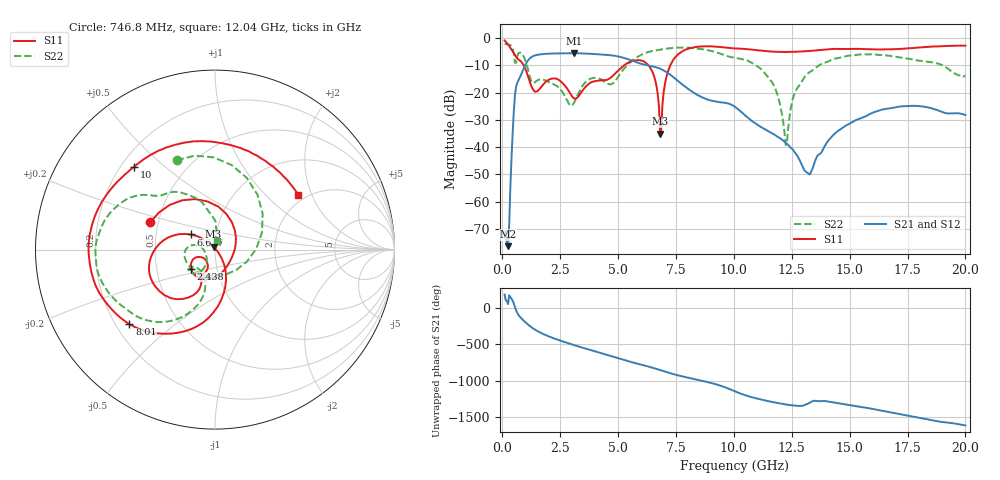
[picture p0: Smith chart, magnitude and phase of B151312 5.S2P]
!  2-Port S-parameters saved by WinCal
! VAR MeasName=S-Parameters (CALIBRATED_DATA) read from VNA (N5244A)
! VAR MeasDate=12/8/2015 5:44:08 PM
! VAR NAME=B151312 5
! VAR FILENAME=B151312 5.S2P
! VAR DATE=12/8/2015 5:44:08 PM
! VAR PHYS_PORTS=1,2
# Hz S DB R 50
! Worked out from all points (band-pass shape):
!   401 points, 100 MHz to 20 GHz, reference 50 ohm
!   highest |S21| = -5.55 dB at 3.085 GHz (marker M1); lowest = -76.4 dB at 249.2 MHz (marker M2)
!   |S21| within 3 dB of the highest: 1.086 GHz to 5.687 GHz (4.601 GHz wide, 136 % of centre)
!   lowest |S11| = -35.2 dB at 6.816 GHz (marker M3), VSWR 1.04, Z = 49.2 + j1.54 ohm
!   |S11| at or under -10 dB: 920.3 MHz to 5.269 GHz (4.349 GHz wide, 141 % of centre); 6.307 GHz to 7.259 GHz (951.8 MHz wide, 14 % of centre)
!   |S22| runs from -39.3 to -2.2 dB; largest |S21 - S12| = 0.0014
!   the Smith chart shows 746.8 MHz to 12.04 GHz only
!   S11 on the Smith chart (normalised r, x): 746.8 MHz: 0.45, +0.16; 2.438 GHz: 0.75, -0.16; 6.617 GHz: 0.75, +0.13; 8.01 GHz: 0.26, -0.35; 10 GHz: 0.25, +0.40; 12.04 GHz: 1.82, +1.60
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1e8  -0.91 -41.8  -73.20 176.7  -81.41 160.5  -2.19 169.3
2.4925e8  -2.42 -93.0  -76.37 46.1  -77.94 66.1  -2.36 152.1
4.98e8  -5.54 -157.8  -26.78 53.0  -26.77 53.0  -5.56 108.2
7.4675e8  -8.15 157.0  -14.71 -121.7  -14.71 -121.7  -5.33 113.2
1.34375e9  -19.11 2.1  -6.61 71.7  -6.61 71.7  -16.58 -89.9
2.43825e9  -15.36 -141.7  -5.65 -84.6  -5.64 -84.6  -18.20 168.3
3.085e9  -22.10 -142.1  -5.55 -151.2  -5.56 -151.2  -23.98 -137.3
3.43325e9  -19.65 -112.4  -5.64 175.0  -5.64 175.0  -17.99 -121.8
4.279e9  -15.57 -121.3  -6.04 96.8  -6.04 96.7  -15.26 -143.7
5.12475e9  -11.02 -115.5  -7.02 17.3  -7.00 17.3  -12.74 -104.1
6.61725e9  -15.92 148.2  -10.69 -113.5  -10.69 -113.6  -4.57 -144.9
6.7665e9  -25.29 132.1  -11.10 -128.2  -11.12 -128.2  -4.34 -149.0
6.81625e9  -35.15 116.4  -11.27 -133.2  -11.29 -133.2  -4.27 -150.4
7.264e9  -9.91 -87.5  -13.55 -177.0  -13.53 -177.0  -3.73 -162.1
8.01025e9  -3.98 -138.9  -18.58 123.0  -18.56 122.9  -3.55 177.7
1.000025e10  -3.81 134.3  -24.97 -57.5  -25.01 -57.7  -7.20 136.7
1.005e10  -3.82 132.4  -25.26 -64.2  -25.29 -64.3  -7.27 136.3
1.204e10  -5.12 33.4  -37.05 128.1  -37.08 128.1  -26.25 73.4
1.228875e10  -5.10 20.1  -38.79 114.9  -38.83 115.2  -38.98 -50.2
1.338325e10  -4.69 -32.2  -48.21 158.7  -48.12 160.7  -11.92 -130.3
1.67165e10  -4.17 -112.1  -25.84 12.5  -25.66 12.3  -6.54 156.1
2e10  -2.83 -147.1  -28.23 -168.9  -28.23 -170.1  -14.09 130.5
